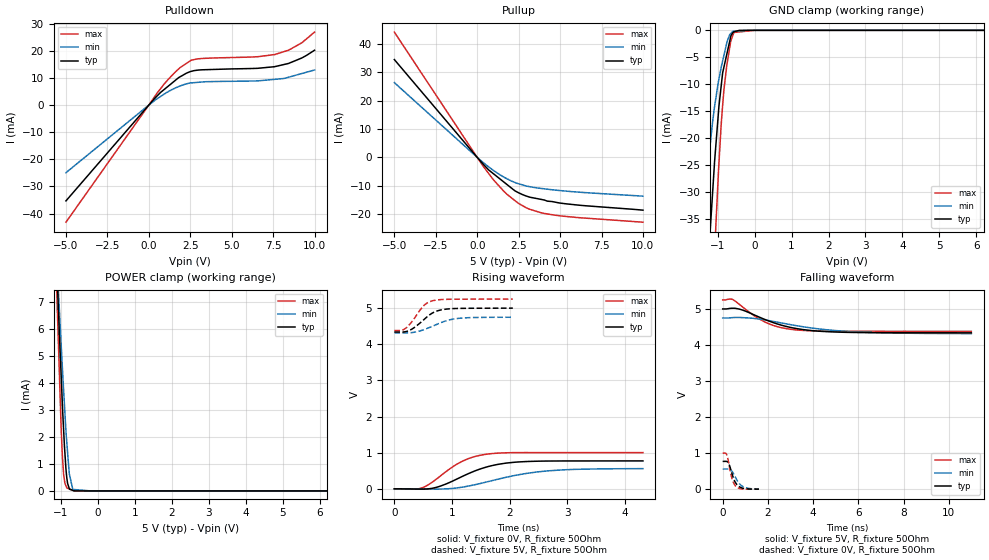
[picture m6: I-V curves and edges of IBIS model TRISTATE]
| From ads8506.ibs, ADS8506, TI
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|   tristate Model
[Model]   TRISTATE
Model_type   3-state
Polarity   Non-Inverting
Vmeas = 2.5
Vref = 2.5
Cref = 10pF
Rref = 50
|   typ   min   max
|   (nom PVT)   (Fast PVT)   (slow PVT)
|C_comp from frequency method(29MHz)
|C_comp   2.989e-12   2.503e-12   3.452e-12
|ON state : BUFFER OUTPUT TURNED HIGH
|C_comp   2.989e-12   2.503e-12   3.452e-12
|OFF state: BUFFER IN HIGH IMPEDANCE
|C_comp   2.847e-12   2.368e-12   3.288e-12
|C_comp from LC tank measurement(L=1nH)
|Resonant Frequency(Hz)   3.420e+09   3.580e+09   3.320e+09
C_comp   2.168e-12   1.978e-12   2.300e-12
|ON state : BUFFER OUTPUT TURNED HIGH
|Resonant Frequency(Hz)   3.420e+09   3.580e+09   3.320e+09
|C_comp   2.168e-12   1.978e-12   2.300e-12
|OFF state: BUFFER IN HIGH IMPEDANCE
|Resonant Frequency(Hz)   3.450e+09   3.640e+09   3.350e+09
|C_comp   2.130e-12   2.259e-12   1.914e-12
| Where nom  PVT is Nominal Process,  5V,  25C
|   Fast PVT is Strong Process,   5.25V,  -40C
|   Slow PVT is Weak Process,   4.75V,  85C
[Voltage Range]   5   4.75   5.25
|Ambient Temperature   25   85   -40
|Junction Temperature
[Temperature Range]   25   85   -40
[Pullup Reference]   5   4.75   5.25
[Pulldown Reference]   0   0   0
[Power Clamp Reference]   5   4.75   5.25
[GND Clamp Reference]   0   0   0
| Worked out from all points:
|   slope of the pulldown table from 0 to 0.75 V, typ, clamps not added: 154 ohm
|   slope of the pullup table from 0 to 0.75 V, typ, clamps not added: 159 ohm
|   GND clamp passes 1 mA (typ) near -0.64 V on its own axis
|   POWER clamp passes 1 mA (typ) near -0.87 V on its own axis
|   falling waveform, V_fixture 5V, R_fixture 50Ohm: 20-80 % time 1.86ns typ, 2.79ns min, 1.36ns max; typ from 5 V to 4.34 V
|   rising waveform, V_fixture 0V, R_fixture 50Ohm: 20-80 % time 706ps typ, 994ps min, 561ps max; typ from 0 V to 0.772 V
|   rising waveform, V_fixture 5V, R_fixture 50Ohm: 20-80 % time 311ps typ, 418ps min, 247ps max; typ from 4.34 V to 5 V
|   falling waveform, V_fixture 0V, R_fixture 50Ohm: 20-80 % time 273ps typ, 337ps min, 220ps max; typ from 0.773 V to 0.004 V
[Pulldown]
|   Voltage   I(typ)   I(min)   I(max)
-5V       -35.3mA    -24.91mA   -43.15mA
255mV     1.772mA    1.23mA     2.249mA
700mV     4.606mA    3.127mA    5.974mA
1.145V    6.828mA    4.861mA    9.3mA
1.906V    10.48mA    7.069mA    13.87mA
2.551V    12.41mA    8.159mA    16.5mA
2.94V     12.86mA    8.357mA    17.01mA
6.557V    13.54mA    8.897mA    17.81mA
7.591V    14.14mA    9.471mA    18.6mA
8.442V    15.36mA    10.27mA    20.24mA
9.229V    17.34mA    11.61mA    22.94mA
10V       20.2mA     12.92mA    26.88mA
[GND Clamp]
|   Voltage   I(typ)   I(min)   I(max)
-5V       -570.3mA   -418.7mA   -735.8mA
-1.49V    -70.85mA   -41.76mA   -110.6mA
-1.31V    -48.88mA   -28.07mA   -78.98mA
-1.171V   -33.84mA   -19.2mA    -55.56mA
-1.055V   -21.93mA   -12.9mA    -37.28mA
-965mV    -14.07mA   -9.031mA   -24.68mA
-903mV    -10.24mA   -6.844mA   -17.38mA
-834.7mV  -6.967mA   -4.783mA   -11.32mA
-750.8mV  -4.385mA   -2.282mA   -6.42mA
-589mV    -446.4uA   -191.3uA   -924.3uA
0V        0A         0A         0A
10V       0A         0A         0A
[Pullup]
|   Voltage   I(typ)   I(min)   I(max)
-5V       34.55mA    26.4mA     44.26mA
362.3mV   -2.4mA     -1.836mA   -3.15mA
700mV     -4.486mA   -3.385mA   -5.78mA
987mV     -5.823mA   -4.656mA   -7.975mA
1.596V    -8.661mA   -6.936mA   -11.91mA
2.27V     -11.8mA    -8.867mA   -15.25mA
2.473V    -12.44mA   -9.281mA   -16.18mA
3.134V    -14mA      -10.32mA   -18.27mA
3.838V    -14.83mA   -10.96mA   -19.55mA
4.508V    -15.6mA    -11.45mA   -20.26mA
6.075V    -16.86mA   -12.27mA   -21.27mA
10V       -18.65mA   -13.7mA    -22.9mA
[POWER Clamp]
|   Voltage   I(typ)   I(min)   I(max)
-5V       62.08mA    56.42mA    69.46mA
-1.306V   15.4mA     14.17mA    16.69mA
-1.097V   7.767mA    8.22mA     6.695mA
-1.085V   7.32mA     7.882mA    6.177mA
-1.045V   5.925mA    6.788mA    4.487mA
-992.2mV  4.226mA    5.379mA    2.293mA
-960.7mV  3.212mA    4.562mA    1.315mA
-924mV    2.182mA    3.656mA    581.2uA
-855mV    676.4uA    2.038mA    162.5uA
-774.2mV  84.76uA    640.5uA    74.31uA
-640.5mV  1.256uA    51.7uA     235nA
10V       0A         0A         0A
[Ramp]
R_load = 50
|   typ   min   max
dV/dt_r   0.464115/7.06943e-10   0.336761/9.96189e-10   0.601524/5.61061e-10
dV/dt_f   0.397163/1.86179e-09   0.260088/2.78889e-09   0.522521/1.35316e-09
[Falling Waveform]
V_fixture = 5V
V_fixture_min = 4.75V
V_fixture_max = 5.25V
R_fixture = 50Ohm
|   Time   V(typ)   V(min)   V(max)
0s        5V         4.75V      5.25V
432ps     5.019V     4.76V      5.264V
885ps     4.968V     4.759V     5.052V
1.365ns   4.843V     4.739V     4.824V
1.818ns   4.721V     4.701V     4.654V
2.391ns   4.589V     4.636V     4.513V
3.045ns   4.482V     4.56V      4.433V
4.167ns   4.388V     4.453V     4.389V
5.907ns   4.347V     4.364V     4.38V
11ns      4.338V     4.317V     4.379V
[Rising Waveform]
V_fixture = 0V
V_fixture_min = 0V
V_fixture_max = 0V
R_fixture = 50Ohm
|   Time   V(typ)   V(min)   V(max)
0s        1.105nV    1.151nV    1.074nV
360ps     -5.463mV   -1.693mV   -9.035mV
489ps     -7.886mV   -3.534mV   32.57mV
786ps     68.7mV     -5.851mV   339mV
1.179ns   343.5mV    46.76mV    762.7mV
1.383ns   487.1mV    108.9mV    887.9mV
1.602ns   605mV      190.7mV    959.4mV
2.028ns   727.2mV    350.2mV    1V
2.685ns   769.1mV    499.7mV    1.002V
4.311ns   772.2mV    559mV      1.002V
[Rising Waveform]
V_fixture = 5V
V_fixture_min = 4.75V
V_fixture_max = 5.25V
R_fixture = 50Ohm
|   Time   V(typ)   V(min)   V(max)
0s        4.338V     4.315V     4.379V
126ps     4.338V     4.315V     4.386V
204ps     4.351V     4.315V     4.451V
333ps     4.447V     4.329V     4.685V
492ps     4.651V     4.392V     5.038V
570ps     4.761V     4.438V     5.142V
651ps     4.854V     4.492V     5.197V
822ps     4.953V     4.605V     5.236V
1.125ns   4.991V     4.717V     5.246V
2.055ns   4.998V     4.747V     5.25V
[Falling Waveform]
V_fixture = 0V
V_fixture_min = 0V
V_fixture_max = 0V
R_fixture = 50Ohm
|   Time   V(typ)   V(min)   V(max)
0s        773.1mV    561.6mV    1.002V
129ps     773.9mV    561.6mV    998.7mV
177ps     771.3mV    562mV      957.2mV
282ps     687.5mV    558.4mV    681.2mV
402ps     453.3mV    504.9mV    317.2mV
495ps     276.3mV    413.1mV    162.3mV
585ps     166.1mV    304.6mV    79.63mV
732ps     72.19mV    158.3mV    24.11mV
897ps     27.59mV    74.85mV    7.615mV
1.602ns   3.622mV    5.232mV    3.114mV
